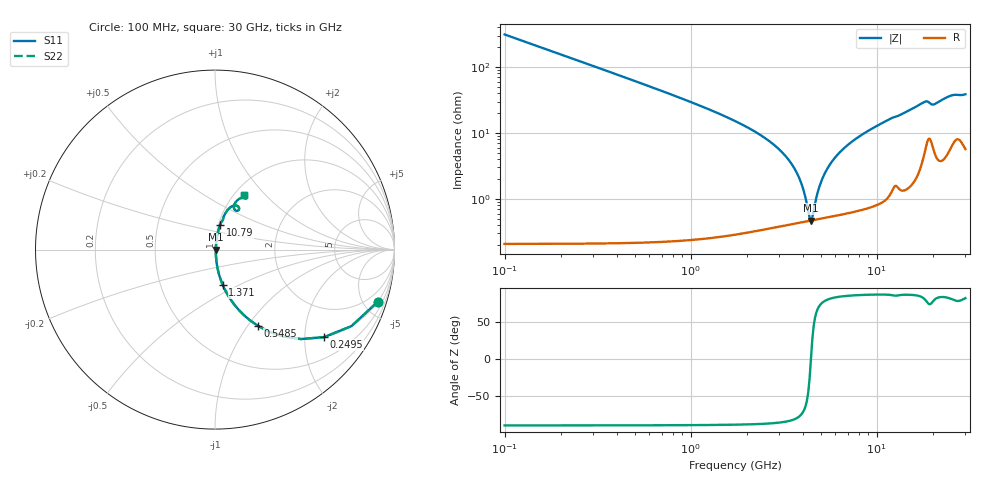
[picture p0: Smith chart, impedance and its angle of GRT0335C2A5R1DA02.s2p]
!Murata Part Number: GRT0335C2A5R1DA02
!These Parameters are Measured in Series Mode Connection
!Data Generated on Jun 19, 2026
!  o--ll--o
!Port1  Port2
!  o------o
!Operation Temp=25[degC], DC Bias Voltage=0[V]
!Freq. Start=100[MHz] Stop=30[GHz] 401[Steps]
# Hz S RI R 50
!Freq.(Hz) S11(Real) S11(Imag) S21(Real) S21(Imag) S12(Real) S12(Imag) S22(Real) S22(Imag)
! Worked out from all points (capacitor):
!   401 points, 100 MHz to 30 GHz, reference 50 ohm
!   read as one part in series: C = 5.1 pF near 249.5 MHz
!   lowest |Z| = 471 mohm at 4.436 GHz (marker M1)
!   series resonance near 4.435 GHz, so ESL is about 250 pH
!   S11 on the Smith chart (normalised r, x): 100 MHz: 1.00, -6.24; 249.5 MHz: 1.00, -2.49; 548.5 MHz: 1.00, -1.12; 1.371 GHz: 1.01, -0.41; 10.79 GHz: 1.02, +0.29; 30 GHz: 1.11, +0.77
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1e8  0.9066 -0.2906  0.0934 0.2906  0.0934 0.2906  0.9066 -0.2906
2.495e8  0.6083 -0.4873  0.3917 0.4873  0.3917 0.4873  0.6083 -0.4873
3.99e8  0.3759 -0.483  0.6241 0.483  0.6241 0.483  0.3759 -0.483
5.485e8  0.2396 -0.4249  0.7604 0.4249  0.7604 0.4249  0.2396 -0.4249
8.475e8  0.1131 -0.3135  0.8869 0.3135  0.8869 0.3135  0.1131 -0.3135
1.37075e9  0.0427 -0.196  0.9573 0.196  0.9573 0.196  0.0427 -0.196
3.46375e9  0.0053 -0.0345  0.9947 0.0345  0.9947 0.0345  0.0053 -0.0345
3.91225e9  0.00469 -0.0173  0.9953 0.0173  0.9953 0.0173  0.00469 -0.0173
4.286e9  0.00463 -0.00472  0.9954 0.00472  0.9954 0.00472  0.00463 -0.00472
4.4355e9  0.00469 6.9e-06  0.9953 -6.9e-06  0.9953 -6.9e-06  0.00469 6.9e-06
4.585e9  0.00479 0.00457  0.9952 -0.00457  0.9952 -0.00457  0.00479 0.00457
4.884e9  0.00511 0.0133  0.9949 -0.0133  0.9949 -0.0133  0.00511 0.0133
5.10825e9  0.00543 0.0195  0.9946 -0.0195  0.9946 -0.0195  0.00543 0.0195
5.781e9  0.00676 0.0368  0.9932 -0.0368  0.9932 -0.0368  0.00676 0.0368
6.75275e9  0.00944 0.0593  0.9906 -0.0593  0.9906 -0.0593  0.00944 0.0593
1.01165e10  0.0242 0.1255  0.9758 -0.1255  0.9758 -0.1255  0.0242 0.1255
1.078925e10  0.0284 0.1377  0.9716 -0.1377  0.9716 -0.1377  0.0284 0.1377
1.505e10  0.06 0.2058  0.94 -0.2058  0.94 -0.2058  0.06 0.2058
1.811475e10  0.1167 0.246  0.8833 -0.246  0.8833 -0.246  0.1167 0.246
2.005825e10  0.1114 0.2203  0.8886 -0.2203  0.8886 -0.2203  0.1114 0.2203
2.50665e10  0.1559 0.2901  0.8441 -0.2901  0.8441 -0.2901  0.1559 0.2901
3e10  0.1634 0.3028  0.8366 -0.3028  0.8366 -0.3028  0.1634 0.3028
